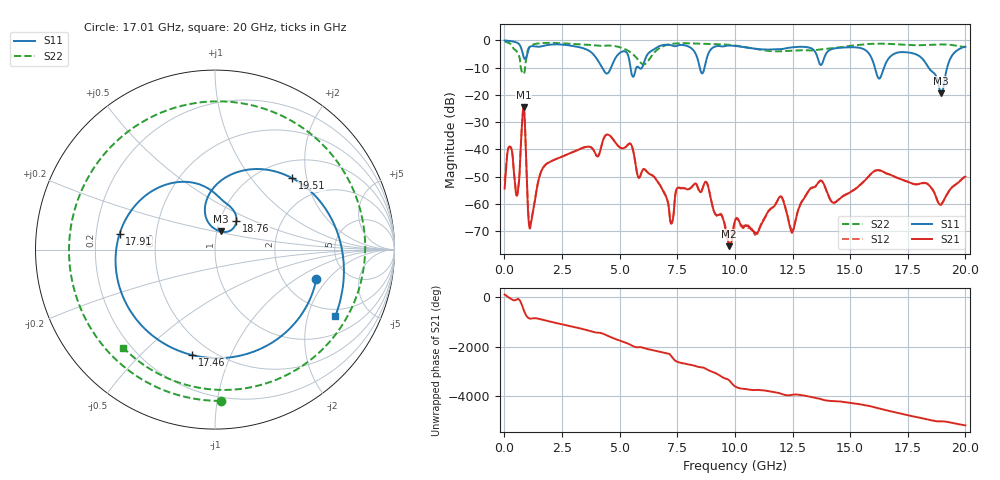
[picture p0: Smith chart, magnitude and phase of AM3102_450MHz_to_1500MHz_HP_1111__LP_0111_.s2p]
!Agilent Technologies,E8364B,MY43040894,A.07.50.67
!Agilent E8364B: A.07.50.67
!Date: Thursday, January 11, 2018 06:50:21
!Correction: S11(Full 2 Port(1,2))
!S21(Full 2 Port(1,2))
!S12(Full 2 Port(1,2))
!S22(Full 2 Port(1,2))
!S2P File: Measurements: S11, S21, S12, S22:
# Hz S  dB  R 50
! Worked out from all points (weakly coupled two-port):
!   1601 points, 10 MHz to 20 GHz, reference 50 ohm
!   highest |S21| = -24.46 dB at 834.6 MHz (marker M1); lowest = -75.6 dB at 9.743 GHz (marker M2)
!   lowest |S11| = -19.5 dB at 18.95 GHz (marker M3), VSWR 1.24, Z = 52.1 + j10.7 ohm
!   |S11| at or under -10 dB: 4.24 GHz to 4.628 GHz (387.5 MHz wide, 8.74 % of centre); 16.07 GHz to 16.47 GHz (396.6 MHz wide, 2.44 % of centre); 18.4 GHz to 19.21 GHz (808.7 MHz wide, 4.3 % of centre)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
!   |S22| runs from -12.3 to -0.4 dB; largest |S21 - S12| = 0.0015
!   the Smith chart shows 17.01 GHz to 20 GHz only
!   S11 on the Smith chart (normalised r, x): 17.01 GHz: 3.02, -1.52; 17.46 GHz: 0.39, -0.73; 17.91 GHz: 0.30, +0.07; 18.76 GHz: 1.20, +0.40; 19.51 GHz: 1.36, +1.65; 20 GHz: 1.68, -3.01
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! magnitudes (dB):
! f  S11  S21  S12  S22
! 10 MHz  -0.1  -54.5  -51.5  -0.4
! 247.4 MHz  -0.3  -39.0  -39.1  -1.2
! 559.7 MHz  -0.9  -56.8  -56.7  -4.4
! 834.6 MHz  -6.2  -24.5  -24.5  -12.3
! 1.134 GHz  -2.2  -68.4  -67.0  -2.0
! 1.709 GHz  -2.0  -46.4  -46.5  -1.0
! 3.346 GHz  -2.7  -39.6  -39.6  -1.5
! 6.682 GHz  -2.3  -52.2  -52.2  -3.1
! 7.256 GHz  -1.9  -67.2  -67.2  -1.3
! 8.756 GHz  -7.3  -52.0  -52.0  -1.3
! 9.743 GHz  -1.9  -75.6  -74.5  -1.6
! 10.01 GHz  -2.1  -66.4  -66.0  -1.9
! 12.49 GHz  -2.6  -70.5  -69.6  -3.8
! 13.34 GHz  -3.1  -54.2  -54.0  -3.7
! 16.68 GHz  -6.6  -49.1  -49.2  -1.3
! 17.01 GHz  -4.6  -50.4  -50.4  -1.5
! 17.46 GHz  -4.4  -51.9  -51.8  -1.7
! 17.91 GHz  -5.4  -52.8  -52.9  -1.8
! 18.76 GHz  -13.9  -58.4  -58.4  -1.6
! 18.95 GHz  -19.5  -60.2  -60.3  -1.5
! 19.51 GHz  -4.6  -53.3  -53.3  -1.8
! 20 GHz  -2.3  -50.0  -50.1  -2.5
